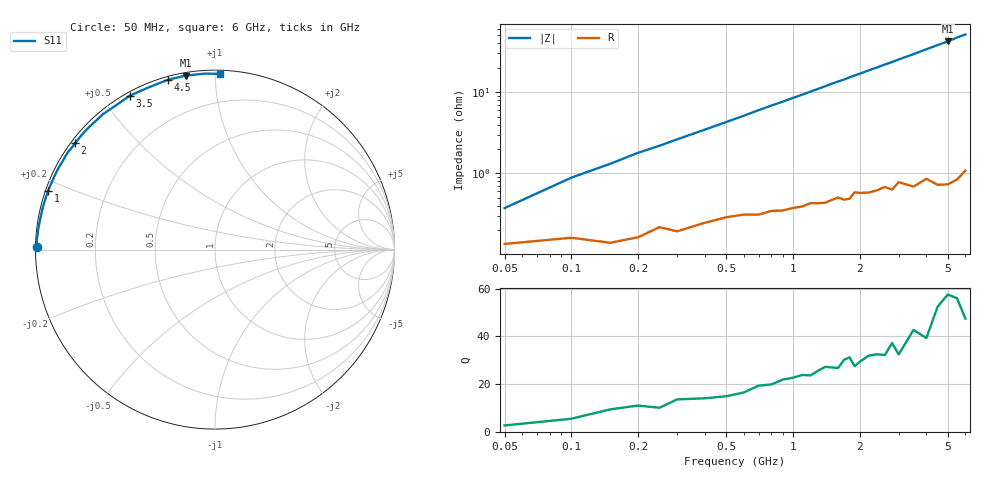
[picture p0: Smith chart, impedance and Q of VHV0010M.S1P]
! Infineon Technologies  Discrete & RF Semiconductors
! BB 814
! Si Tuning Diode in SOT23
! VR =
! S-Parameters:  July  1999
# GHz  S  MA  R  50
!  f  S11
! GHz  MAG  ANG
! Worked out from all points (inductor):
!   34 points, 50 MHz to 6 GHz, reference 50 ohm
!   read as one part to ground: L = 1.39 nH near 100 MHz
!   highest Q = 56 at 5 GHz (marker M1), where L = 1.34 nH
!   S11 on the Smith chart (normalised r, x): 50 MHz: 0.00, +0.01; 1 GHz: 0.01, +0.17; 2 GHz: 0.01, +0.34; 3.5 GHz: 0.01, +0.59; 4.5 GHz: 0.01, +0.76; 6 GHz: 0.02, +1.03
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0.05  0.9946 179.2
0.1  0.9936 178.0
0.2  0.9935 175.9
0.25  0.9913 175.0
0.3  0.9923 174.0
0.6  0.9877 168.3
0.7  0.9878 166.3
0.8  0.9865 164.4
1  0.9855 160.7
1.1  0.985 158.9
1.3  0.9838 155.2
1.5  0.9824 151.4
1.6  0.9813 149.7
1.7  0.9826 148.0
1.8  0.9823 146.1
1.9  0.979 144.3
2  0.9795 142.7
2.2  0.9798 139.2
2.4  0.9788 136.0
2.6  0.9774 132.6
2.8  0.9795 129.6
3  0.9755 126.3
3.5  0.9797 119.0
4  0.9767 111.9
4.5  0.9818 105.4
5  0.983 99.6
5.5  0.9823 93.3
6  0.9791 88.4
